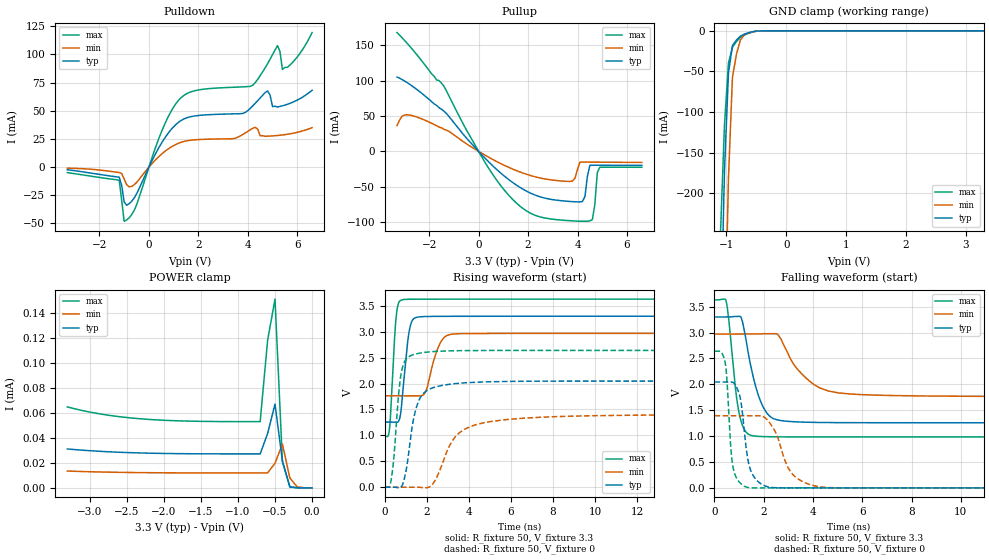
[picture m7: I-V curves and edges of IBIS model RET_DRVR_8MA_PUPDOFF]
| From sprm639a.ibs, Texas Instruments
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|   Model Cell RET_DRVR_8MA_PUPDOFF
|RET_DRVR_8MA_PUPDOFF
[Model]   RET_DRVR_8MA_PUPDOFF
Model_type   I/O
Polarity   Non-Inverting
Enable   Active-Low
Vinl =  0.8
Vinh =  2
Cref =  15.0000pF
Rref =  100.0000M
Vref =  0V
Vmeas =  1.65
C_comp   5.345208p   4.561426p   6.022817p
[Model Spec]
Vinl   0.8   0.8   0.8
Vinh   2   2   2
[Temperature Range]   25   155   -40
[Voltage Range]   3.3   2.97   3.63
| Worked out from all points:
|   slope of the pulldown table from 0 to 0.495 V, typ, clamps not added: 23.8 ohm
|   slope of the pullup table from 0 to 0.495 V, typ, clamps not added: 27.8 ohm
|   GND clamp passes 1 mA (typ) near -0.55 V on its own axis
|   rising waveform, R_fixture 50, V_fixture 3.3: 20-80 % time 297ps typ, 507ps min, 211ps max; typ from 1.26 V to 3.3 V
|   rising waveform, R_fixture 50, V_fixture 0: 20-80 % time 533ps typ, 1.22ns min, 323ps max; typ from 0 V to 2.04 V
|   falling waveform, R_fixture 50, V_fixture 3.3: 20-80 % time 607ps typ, 1.17ns min, 363ps max; typ from 3.3 V to 1.26 V
|   falling waveform, R_fixture 50, V_fixture 0: 20-80 % time 337ps typ, 712ps min, 210ps max; typ from 2.04 V to 0 V
| Nom Voltages:
|   BIASFET=3.3, VDD=1.2, VDDS=3.3, VSS=0
| Min Voltages:
|   BIASFET=2.97, VDD=1.08, VDDS=2.97, VSS=0
| Max Voltages:
|   BIASFET=3.63, VDD=1.32, VDDS=3.63, VSS=0
[POWER_clamp]
|   voltage   I(typ)   I(min)   I(max)
-3.3V     31.22uA    13.5uA     64.95uA
-2.8V     29.13uA    12.67uA    58.77uA
-2.3V     27.98uA    12.22uA    55.36uA
-1.7V     27.4uA     12.01uA    53.62uA
-700mV    27.24uA    11.95uA    53.12uA
-600mV    43.52uA    11.94uA    118.2uA
-500mV    67.2uA     19.79uA    151.5uA
-400mV    21.58uA    35.09uA    21.1uA
-300mV    927.4nA    7.958uA    611.4nA
-200mV    28.93nA    716.3nA    11.51nA
0V        696.9pA    39.48nA    568pA
[Pulldown]
|   voltage   I(typ)   I(min)   I(max)
-3.3V     -2.325mA   -885.1uA   -4.829mA
-1.2V     -8.9mA     -4.742mA   -11.78mA
-1V       -30.94mA   -10.56mA   -48.07mA
-900mV    -33.77mA   -15.53mA   -46.9mA
-500mV    -23.82mA   -13.61mA   -33.55mA
600mV     24.46mA    13.16mA    36.18mA
1.3V      41.39mA    22.04mA    61.62mA
4.2V      54.39mA    34.49mA    72.77mA
4.8V      67.66mA    27.49mA    91.8mA
5.2V      53.41mA    28.11mA    107.8mA
5.4V      54.46mA    28.58mA    86.79mA
6.6V      68.25mA    35.07mA    119.5mA
[Pullup]
|   voltage   I(typ)   I(min)   I(max)
-3.3V     105mA      36.43mA    167.7mA
-2.4V     84.74mA    47.23mA    132.2mA
-1.4V     56.66mA    31.22mA    91.73mA
700mV     -24.56mA   -13.78mA   -39.08mA
2.1V      -58.93mA   -34.12mA   -87.33mA
3.8V      -70.97mA   -41.82mA   -98.09mA
4.2V      -70.71mA   -15.14mA   -98.64mA
4.5V      -19.61mA   -15.2mA    -98.06mA
4.6V      -19.61mA   -15.22mA   -96.39mA
4.8V      -19.61mA   -15.26mA   -30.07mA
4.9V      -19.62mA   -15.28mA   -22.42mA
6.6V      -19.78mA   -15.6mA    -22.44mA
[GND_clamp]
|   voltage   I(typ)   I(min)   I(max)
-3.3V     -16.36A    -15.08A    -17.18A
-1.1V     -382.1mA   -717.8mA   -250.1mA
-1.033V   -173.3mA   -402.2mA   -116.4mA
-966.7mV  -52.02mA   -182.1mA   -39.81mA
-900mV    -18.21mA   -57.43mA   -20.34mA
-833.3mV  -11.36mA   -28.88mA   -13.17mA
-766.7mV  -6.618mA   -11.27mA   -8.134mA
-700mV    -3.983mA   -4.59mA    -5.247mA
-500mV    -328.3uA   -481.4uA   -374.5uA
-366.7mV  -15.94uA   -50.74uA   -14.83uA
3.3V      696.9pA    15.84uA    426.1pA
[Ramp]
| variable   typ   min   max
dV/dt_f  1.2327083/0.6089555n 0.72801541/1.1737387n   1.597487/0.3638698n
dV/dt_r  1.2367288/0.5366087n  0.8469789/1.2334714n  1.5908665/0.32475913n
R_load = 50
[Rising Waveform]
R_fixture = 50
V_fixture = 3.3
V_fixture_min = 2.97
V_fixture_max = 3.63
|   time   V(typ)   V(min)   V(max)
0s        1.258V     1.765V     982mV
224.7ps   1.258V     1.765V     1.121V
543.4ps   1.253V     1.765V     3.298V
790.9ps   1.546V     1.765V     3.613V
1.139ns   2.958V     1.765V     3.628V
1.502ns   3.278V     1.765V     3.629V
1.938ns   3.295V     1.841V     3.629V
2.552ns   3.298V     2.709V     3.63V
3.132ns   3.299V     2.95V      3.63V
20.01ns   3.3V       2.97V      3.63V
[Rising Waveform]
R_fixture = 50
V_fixture = 0
V_fixture_min = 0
V_fixture_max = 0
|   time   V(typ)   V(min)   V(max)
0s        0V         0V         0V
325.3ps   0V         0V         193.9mV
684.5ps   -12.21mV   0V         1.908V
854.8ps   61.54mV    0V         2.331V
1.309ns   1.189V     0V         2.552V
1.617ns   1.671V     0V         2.585V
1.98ns    1.859V     -10.8mV    2.606V
3.375ns   2V         984.5mV    2.634V
4.713ns   2.032V     1.243V     2.639V
20.2ns    2.045V     1.397V     2.639V
[Falling Waveform]
R_fixture = 50
V_fixture = 3.3
V_fixture_min = 2.97
V_fixture_max = 3.63
|   time   V(typ)   V(min)   V(max)
0s        3.3V       2.97V      3.63V
468.7ps   3.3V       2.97V      3.613V
956.5ps   3.311V     2.97V      1.555V
1.14ns    3.202V     2.97V      1.201V
1.441ns   2.428V     2.97V      1.019V
1.983ns   1.554V     2.977V     990.1mV
2.772ns   1.294V     2.796V     984.4mV
3.81ns    1.267V     2.081V     982.9mV
5.03ns    1.26V      1.834V     982.7mV
20.01ns   1.258V     1.765V     982.8mV
[Falling Waveform]
R_fixture = 50
V_fixture = 0
V_fixture_min = 0
V_fixture_max = 0
|   time   V(typ)   V(min)   V(max)
0s        2.045V     1.393V     2.639V
438.7ps   2.045V     1.393V     2.408V
692.2ps   2.046V     1.393V     609.6mV
929.8ps   1.911V     1.393V     161.8mV
1.091ns   1.613V     1.393V     70.54mV
1.329ns   624.4mV    1.393V     8.933mV
2.024ns   41.84mV    1.365V     0V
3.073ns   0V         321.8mV    0V
4.149ns   0V         30.31mV    0V
20.2ns    0V         0V         0V
